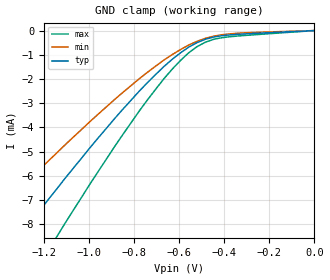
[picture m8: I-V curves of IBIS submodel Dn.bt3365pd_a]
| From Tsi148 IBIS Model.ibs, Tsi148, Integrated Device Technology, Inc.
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[Submodel]  Dn.bt3365pd_a
Submodel_type   Dynamic_clamp
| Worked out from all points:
|   GND clamp passes 1 mA (typ) near -0.61 V on its own axis
[GND Clamp]   | Note: Vtable =  Vout
| Voltage   I(typ)   I(min)   I(max)
-3.6V     -38.58mA   -29.75mA   -48.66mA
-1.51V    -10.99mA   -8.444mA   -14.16mA
-1.473V   -10.53mA   -8.096mA   -13.59mA
-1.29V    -8.288mA   -6.384mA   -10.74mA
-1.143V   -6.541mA   -5.053mA   -8.516mA
-1.107V   -6.112mA   -4.727mA   -7.969mA
-777mV    -2.5mA     -1.988mA   -3.321mA
-667mV    -1.479mA   -1.214mA   -1.981mA
-557mV    -680uA     -595uA     -912uA
-483mV    -356uA     -319uA     -477uA
-410mV    -212uA     -171uA     -294uA
0V        0A         0A         0A
